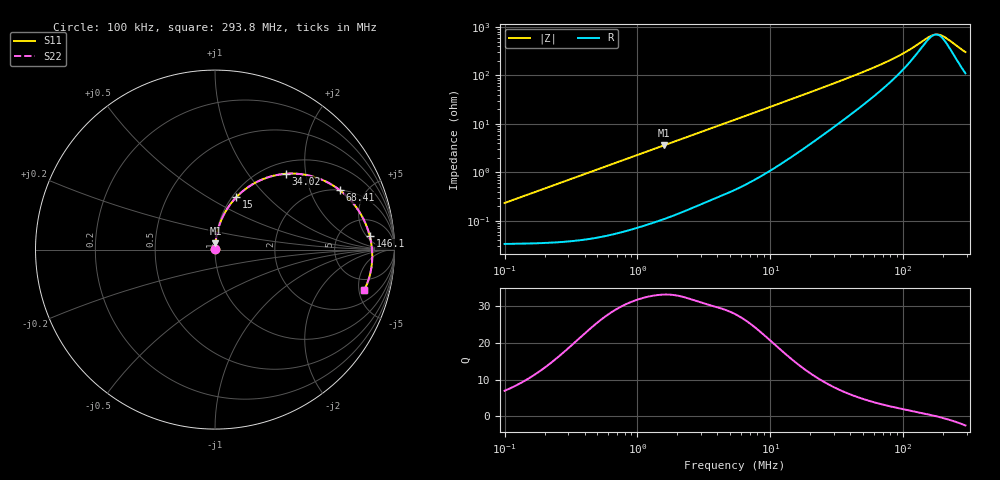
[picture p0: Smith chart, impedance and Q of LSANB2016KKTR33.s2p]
! LSANB2016KKTR33  S-PARAMETER MODEL  ( General Type )
! Model Generated by TAIYO YUDEN Corporation (http://www.ty-top.com)
! Version 2.0
! TAIYO YUDEN Control No. 20210629
! Copyright(c) 2016 TAIYO YUDEN CO.,LTD. All Rights Reserved.
! Product Description (link to TY-COMPAS)
! https://ds.yuden.co.jp/TYCOMPAS/or/detail?pn=LSANB2016KKTR33M&u=M
! Products Name : Inductors
! Characteristics :
!  Inductance : 0.33 uH , SRF(min) : -Hz , DC Resistance(max) : 0.04 Ohm
!  Rated Current : Saturation :3600 mA , Temp Rise : 3200 mA (40 degC)
!  Case Size : 2.0 x 1.6 / 0.079 x 0.063 [mm/inch] , Thickness : 1 / 0.039 [mm/inch]
!  (Conditions: Temperature = 25 degC , DC Bias Current/Voltage = 0A / 0V)
! External Node Assignments :
!  1  o---GGG---o  2
! GND o---------o GND
! Frequency Range : 0.1MHz  -  293.796821MHz  [ 402 STEP ]
# MHz S RI R 50
! Freq[MHz].  S11 Real  S11 Imag  S21 Real  S21 Imag  S12 Real  S12 Imag  S22 Real  S22 Imag
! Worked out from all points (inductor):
!   401 points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, 100 kHz to 293.8 MHz, reference 50 ohm
!   read as one part in series: L = 369 nH near 104.1 kHz
!   highest Q = 33.2 at 1.572 MHz (marker M1), where L = 364 nH
!   self-resonance near 175.2 MHz
!   S11 on the Smith chart (normalised r, x): 100 kHz: 1.00, +0.00; 15 MHz: 1.04, +0.68; 34.02 MHz: 1.22, +1.55; 68.41 MHz: 2.00, +3.26; 146.1 MHz: 10, +6; 293.8 MHz: 3.21, -5.65
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0.1  0.00034 0.00232  0.9997 -0.00232  0.9997 -0.00232  0.00034 0.00232
0.380976  0.000481 0.00881  0.9995 -0.00881  0.9995 -0.00881  0.000481 0.00881
1.451429  0.0021 0.0331  0.9979 -0.0331  0.9979 -0.0331  0.0021 0.0331
1.572086  0.00237 0.0358  0.9976 -0.0358  0.9976 -0.0358  0.00237 0.0358
3.099276  0.00715 0.0696  0.9929 -0.0696  0.9929 -0.0696  0.00715 0.0696
5.420303  0.0189 0.1193  0.9811 -0.1193  0.9811 -0.1193  0.0189 0.1193
9.670679  0.054 0.2036  0.946 -0.2036  0.946 -0.2036  0.054 0.2036
15.00374  0.118 0.2912  0.882 -0.2912  0.882 -0.2912  0.118 0.2912
20.65007  0.1996 0.3581  0.8004 -0.3581  0.8004 -0.3581  0.1996 0.3581
27.30883  0.2997 0.4042  0.7003 -0.4042  0.7003 -0.4042  0.2997 0.4042
34.01531  0.394 0.4223  0.606 -0.4223  0.606 -0.4223  0.394 0.4223
47.76023  0.5489 0.4061  0.4511 -0.4061  0.4511 -0.4061  0.5489 0.4061
68.4114  0.6939 0.3322  0.3061 -0.3322  0.3061 -0.3322  0.6939 0.3322
78.67184  0.7395 0.2921  0.2605 -0.2921  0.2605 -0.2921  0.7395 0.2921
106.138  0.8147 0.193  0.1853 -0.193  0.1853 -0.193  0.8147 0.193
146.0807  0.8626 0.0737  0.1374 -0.0737  0.1374 -0.0737  0.8626 0.0737
167.9901  0.873 0.0175  0.127 -0.0175  0.127 -0.0175  0.873 0.0175
178.3586  0.8753 -0.00739  0.1247 0.00739  0.1247 0.00739  0.8753 -0.00739
189.3671  0.8762 -0.0328  0.1238 0.0328  0.1238 0.0328  0.8762 -0.0328
209.245  0.8744 -0.076  0.1256 0.076  0.1256 0.076  0.8744 -0.076
271.248  0.8466 -0.1919  0.1534 0.1919  0.1534 0.1919  0.8466 -0.1919
293.7968  0.8305 -0.2274  0.1695 0.2274  0.1695 0.2274  0.8305 -0.2274
